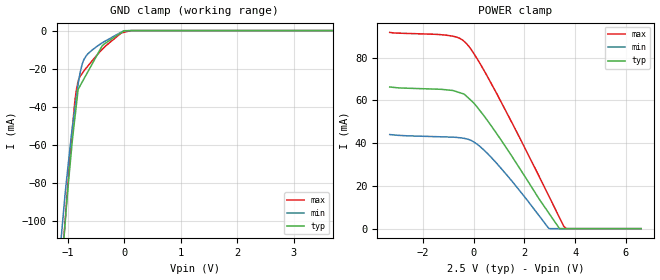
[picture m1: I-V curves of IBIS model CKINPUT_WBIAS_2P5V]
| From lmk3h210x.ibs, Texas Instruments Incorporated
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[Model]   CKINPUT_WBIAS_2P5V
Model_type   Input
Vinl = 0.2
Vinh = 0.4
|   typ   min   max
C_comp   1.5pF   1.4pF   1.6pF
[Voltage Range]   2.5   2.25   2.75
[Temperature Range]   50   125   -40
[Power Clamp Reference]   2.5   2.25   2.75
[GND Clamp Reference]   0   0   0
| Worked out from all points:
|   GND clamp passes 1 mA (typ) near -0.05 V on its own axis
[GND Clamp]
|   Voltage   I(typ)   I(min)   I(max)
-3.3V     -1.023A    -928mA     -1.13A
-1.209V   -162mA     -139.3mA   -169mA
-1.065V   -107.8mA   -91.57mA   -107.2mA
-1.051V   -102.5mA   -86.96mA   -101.7mA
-934.8mV  -62.44mA   -54.38mA   -56.05mA
-877.3mV  -46.53mA   -41.62mA   -37.87mA
-816.2mV  -30.81mA   -28.06mA   -26.49mA
-751.2mV  -27.32mA   -18.29mA   -22.73mA
-668.2mV  -22.87mA   -12.99mA   -19.46mA
-388.1mV  -7.841mA   -6.381mA   -9.788mA
-3.764mV  -73.56uA   -283.4uA   -906.7uA
6.6V      0A         0A         0A
[POWER Clamp]
|   Voltage   I(typ)   I(min)   I(max)
-3.3V     66.27mA    44.03mA    91.82mA
-1.091V   64.99mA    42.91mA    90.53mA
-541.9mV  63.61mA    42.54mA    89.01mA
-271.8mV  61.9mA     41.99mA    86.51mA
207.3mV   55.89mA    38.9mA     78.19mA
858.4mV   45.36mA    31.27mA    64.37mA
1.912V    26.42mA    16.34mA    40.26mA
2.964V    7.29mA     100.4uA    15.3mA
3.386V    0A         0A         5.1mA
3.55V     0A         0A         1.152mA
3.653V    0A         0A         0A
6.6V      0A         0A         0A
